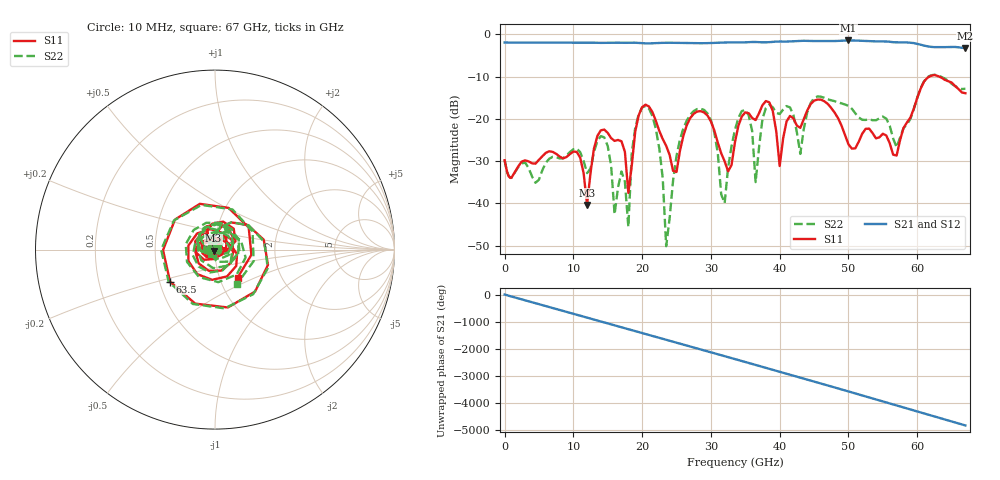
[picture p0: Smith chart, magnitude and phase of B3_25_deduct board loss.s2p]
!Keysight Technologies,N5247B,MY61255065,A.16.20.04
!Date: Monday, September 04, 2023 01:12:37
!Correction: S11(C  2-Port  )
!S21(C  2-Port  )
!S12(C  2-Port  )
!S22(C  2-Port  )
!S2P File: Measurements: S11, S21, S12, S22:
!Deduct Board Loss
# Hz S  dB  R 50
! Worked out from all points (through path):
!   142 points, 10 MHz to 67 GHz, reference 50 ohm
!   highest |S21| = -1.46 dB at 50 GHz (marker M1); lowest = -3.2 dB at 67 GHz (marker M2)
!   lowest |S11| = -40.4 dB at 12 GHz (marker M3), VSWR 1.02, Z = 49.2 - j0.561 ohm
!   |S11| at or under -10 dB: start of sweep to 61.78 GHz; 63.17 GHz to end of sweep
!   |S22| runs from -50.1 to -9.6 dB; largest |S21 - S12| = 0.0036
!   S11 on the Smith chart (normalised r, x): 10 MHz: 0.94, -0.00; 63.5 GHz: 0.57, -0.22; 67 GHz: 1.22, -0.40
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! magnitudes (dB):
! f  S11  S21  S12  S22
! 10 MHz  -29.8  -1.9  -1.9  -29.7
! 11.5 GHz  -32.9  -2.0  -2.0  -30.0
! 12 GHz  -40.4  -2.0  -2.0  -32.9
! 14 GHz  -22.7  -2.0  -2.0  -24.1
! 18 GHz  -37.5  -2.0  -2.0  -45.6
! 19.5 GHz  -19.2  -2.0  -2.0  -19.0
! 22.5 GHz  -22.9  -2.1  -2.1  -27.0
! 23.5 GHz  -26.4  -2.0  -2.0  -50.1
! 26.5 GHz  -21.5  -2.1  -2.1  -20.4
! 30 GHz  -20.6  -2.1  -2.1  -20.3
! 32 GHz  -30.1  -1.9  -1.9  -39.9
! 34 GHz  -21.6  -1.9  -1.9  -19.8
! 35.5 GHz  -18.7  -1.9  -1.9  -19.2
! 36.5 GHz  -20.3  -1.8  -1.8  -35.0
! 38 GHz  -15.8  -1.9  -1.9  -17.4
! 40 GHz  -31.2  -1.7  -1.7  -18.9
! 43 GHz  -22.1  -1.5  -1.5  -28.3
! 45 GHz  -15.7  -1.6  -1.6  -15.1
! 50 GHz  -26.0  -1.5  -1.5  -16.9
! 56 GHz  -25.8  -1.8  -1.8  -21.6
! 63.5 GHz  -10.2  -3.0  -3.0  -10.1
! 67 GHz  -13.9  -3.2  -3.2  -12.9
